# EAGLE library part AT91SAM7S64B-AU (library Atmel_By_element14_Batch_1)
AT91 ARM Thumb-based Microcontrollers
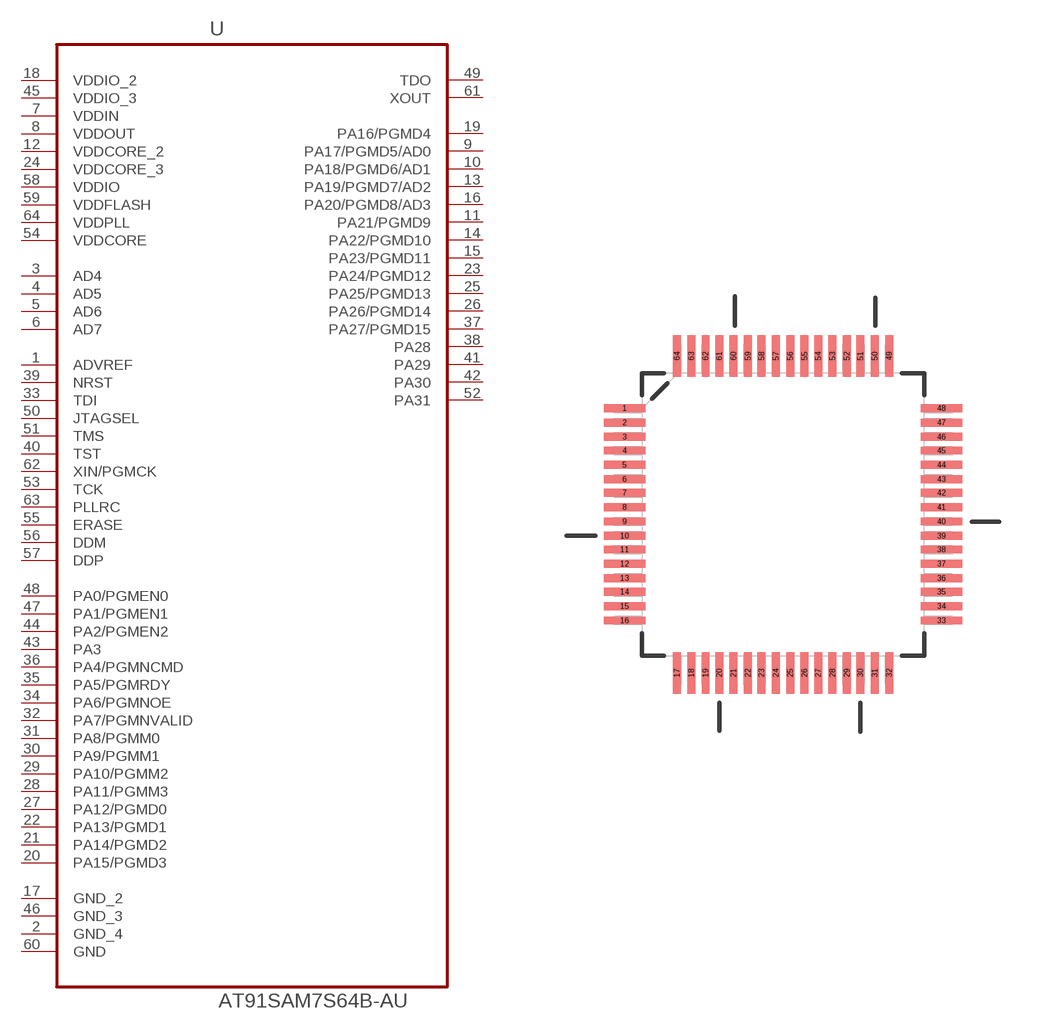
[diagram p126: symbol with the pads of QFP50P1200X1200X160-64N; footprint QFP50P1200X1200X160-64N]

Designator prefix U

## AT91SAM7S64B-AU (DESCRIPTION: AT91 ARM Thumb-based Microcontrollers; MPN: AT91SAM7S64B-AU; OC_FARNELL: 1699393; OC_NEWARK: -; PACKAGE: QFP-64; SUPPLIER: Atmel)  [QFP50P1200X1200X160-64N]
1  ADVREF  in
2  GND_4  pas
3  AD4  in
4  AD5  in
5  AD6  in
6  AD7  in
7  VDDIN  pwr
8  VDDOUT  pwr
9  PA17/PGMD5/AD0
10  PA18/PGMD6/AD1
11  PA21/PGMD9
12  VDDCORE_2  pwr
13  PA19/PGMD7/AD2
14  PA22/PGMD10
15  PA23/PGMD11
16  PA20/PGMD8/AD3
17  GND_2  pas
18  VDDIO_2  pwr
19  PA16/PGMD4
20  PA15/PGMD3
21  PA14/PGMD2
22  PA13/PGMD1
23  PA24/PGMD12
24  VDDCORE_3  pwr
25  PA25/PGMD13
26  PA26/PGMD14
27  PA12/PGMD0
28  PA11/PGMM3
29  PA10/PGMM2
30  PA9/PGMM1
31  PA8/PGMM0
32  PA7/PGMNVALID
33  TDI  in
34  PA6/PGMNOE
35  PA5/PGMRDY
36  PA4/PGMNCMD
37  PA27/PGMD15
38  PA28
39  NRST  in
40  TST  in
41  PA29
42  PA30
43  PA3
44  PA2/PGMEN2
45  VDDIO_3  pwr
46  GND_3  pas
47  PA1/PGMEN1
48  PA0/PGMEN0
49  TDO
50  JTAGSEL  pas
51  TMS  in
52  PA31
53  TCK  in
54  VDDCORE  pwr
55  ERASE  in
56  DDM  in
57  DDP  in
58  VDDIO  pwr
59  VDDFLASH  pwr
60  GND  pas
61  XOUT  out
62  XIN/PGMCK  in
63  PLLRC  pas
64  VDDPLL  pwr

## Footprint QFP50P1200X1200X160-64N (pad centres in mm)
smd 1.473 x 0.279: 1 -5.613,3.759; 2 -5.613,3.251; 3 -5.613,2.743; 4 -5.613,2.261; 5 -5.613,1.753; 6 -5.613,1.245; 7 -5.613,0.762; 8 -5.613,0.254; 9 -5.613,-0.254; 10 -5.613,-0.762; 11 -5.613,-1.245; 12 -5.613,-1.753; 13 -5.613,-2.261; 14 -5.613,-2.743; 15 -5.613,-3.251; 16 -5.613,-3.759; 33 5.613,-3.759; 34 5.613,-3.251; 35 5.613,-2.743; 36 5.613,-2.261; 37 5.613,-1.753; 38 5.613,-1.245; 39 5.613,-0.762; 40 5.613,-0.254; 41 5.613,0.254; 42 5.613,0.762; 43 5.613,1.245; 44 5.613,1.753; 45 5.613,2.261; 46 5.613,2.743; 47 5.613,3.251; 48 5.613,3.759
smd 0.279 x 1.473: 17 -3.759,-5.613; 18 -3.251,-5.613; 19 -2.743,-5.613; 20 -2.261,-5.613; 21 -1.753,-5.613; 22 -1.245,-5.613; 23 -0.762,-5.613; 24 -0.254,-5.613; 25 0.254,-5.613; 26 0.762,-5.613; 27 1.245,-5.613; 28 1.753,-5.613; 29 2.261,-5.613; 30 2.743,-5.613; 31 3.251,-5.613; 32 3.759,-5.613; 49 3.759,5.613; 50 3.251,5.613; 51 2.743,5.613; 52 2.261,5.613; 53 1.753,5.613; 54 1.245,5.613; 55 0.762,5.613; 56 0.254,5.613; 57 -0.254,5.613; 58 -0.762,5.613; 59 -1.245,5.613; 60 -1.753,5.613; 61 -2.261,5.613; 62 -2.743,5.613; 63 -3.251,5.613; 64 -3.759,5.613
